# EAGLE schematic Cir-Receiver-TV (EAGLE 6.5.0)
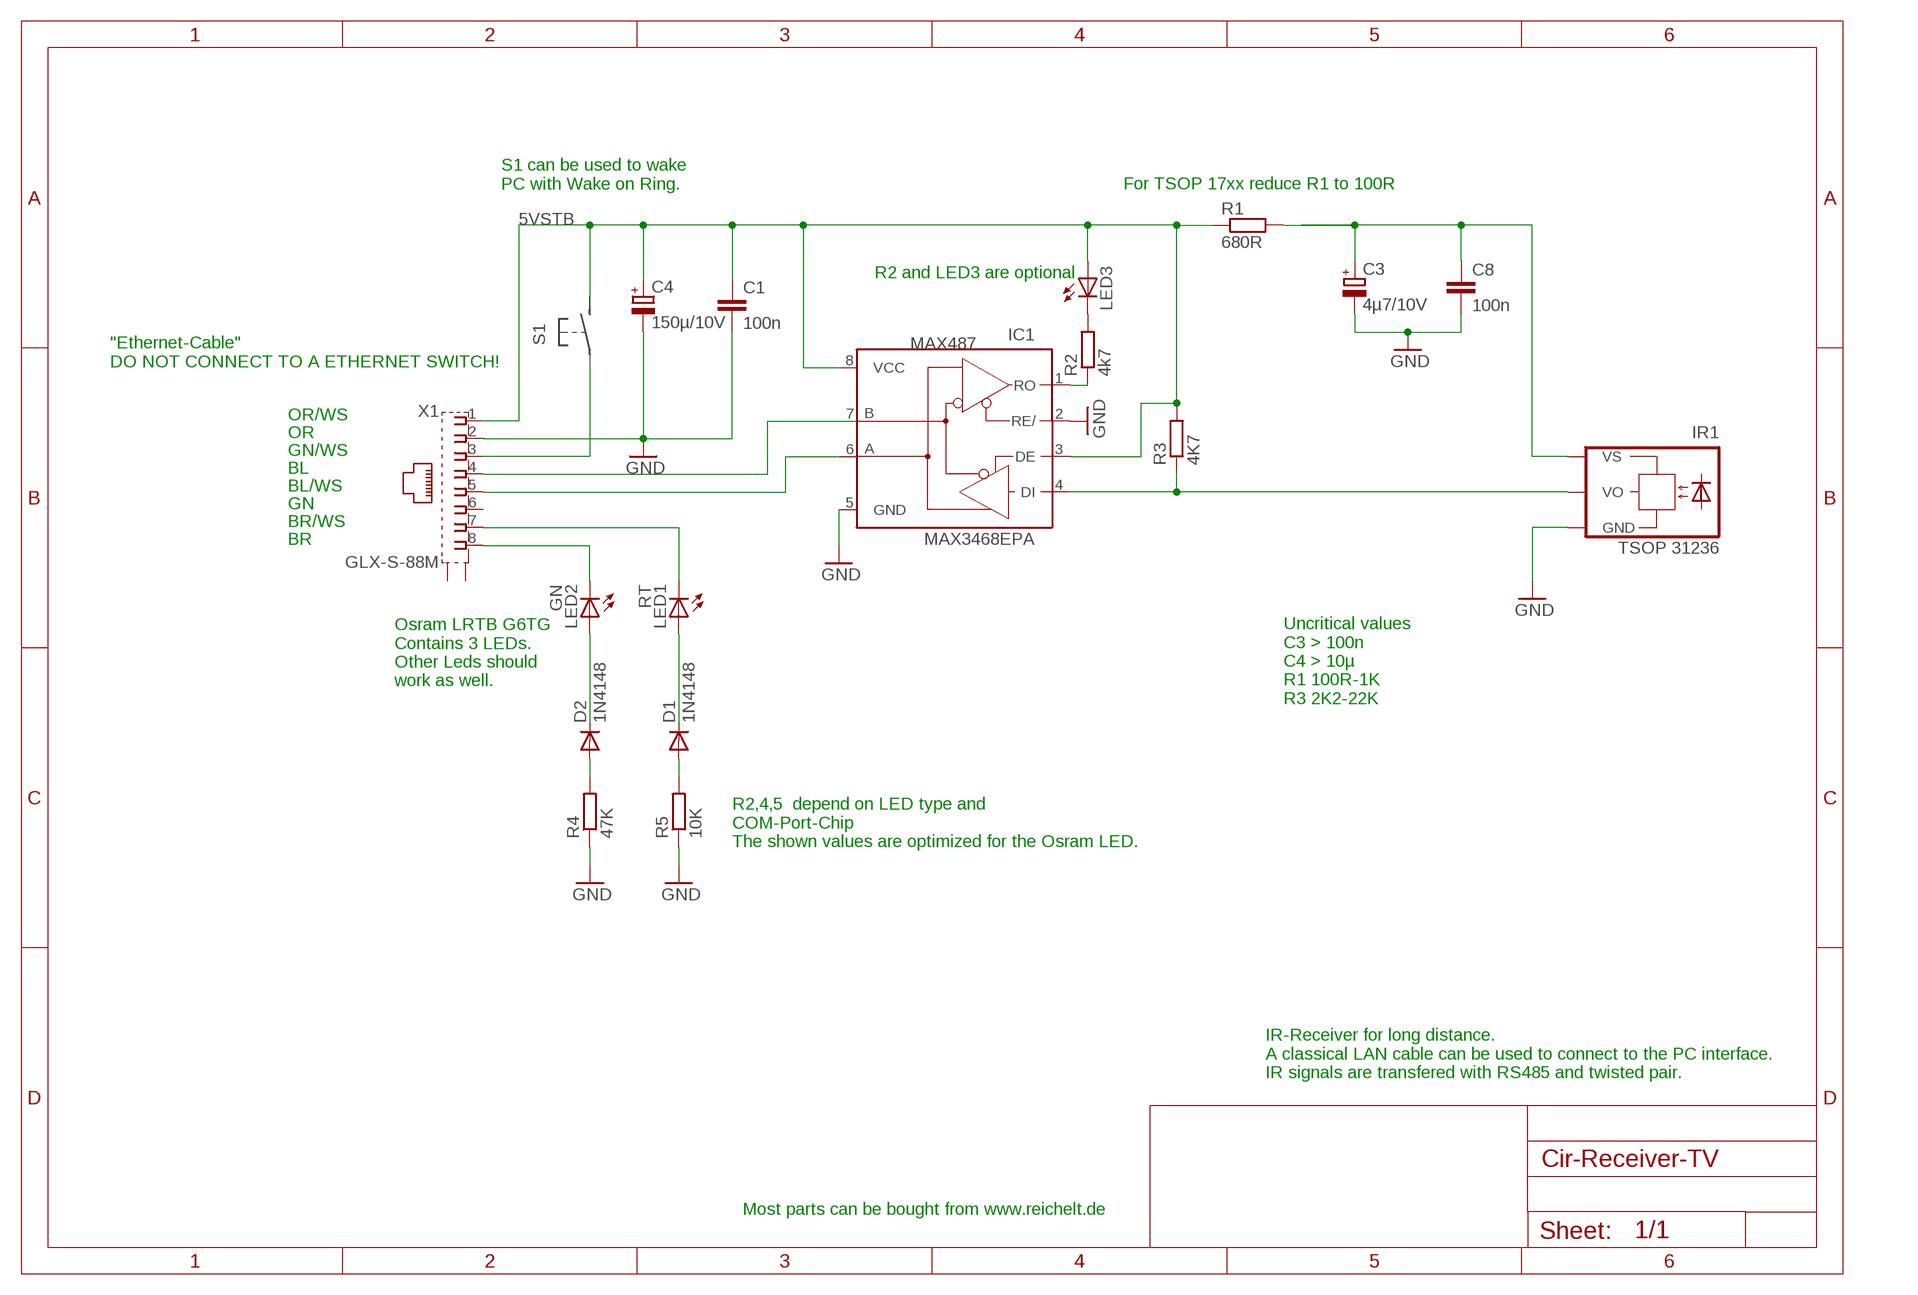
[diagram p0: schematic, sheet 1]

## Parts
C1  100n  C2,5-3  [C2.5-3]
C3  4µ7/10V  CPOL-EUE2.5-5  [E2,5-5]
C4  150µ/10V  CPOL-EUE2.5-5  [E2,5-5]
C8  100n  C2,5-3  [C2.5-3]
D1  1N4148  1N4148DO35-7  [DO35-7]
D2  1N4148  1N4148DO35-7  [DO35-7]
IC1  MAX3468EPA  [DIL08]
IR1  TSOP 31236  TSOP1737TB1  [TSOP17_TB1]
LED1  RT  LED3MM  [LED3MM]
LED2  GN  LED3MM  [LED3MM]
LED3  LED3MM  [LED3MM]
R1  680R  R-EU_0207/10  [0207/10]
R2  4k7  R-EU_0207/10  [0207/10]
R3  4K7  R-EU_0207/10  [0207/10]
R4  47K  R-EU_0207/10  [0207/10]
R5  10K  R-EU_0207/10  [0207/10]
X1  GLX-S-88M  [GLX-S-88M]

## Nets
5VSTB: C1.1 C4.+ IC1.3(DE) IC1.8(VCC) LED3.A R1.1 R3.2 X1.1
GND: C1.2 C3.- C4.- C8.2 IC1.2(RE/) IC1.5(GND) IR1.GND R4.1 R5.1 X1.2
N$1: C3.+ C8.1 IR1.VS R1.2
N$2: IC1.4(DI) IR1.VO R3.1
N$3: X1.3
N$4: LED3.K(C) R2.2
N$5: IC1.1(RO) R2.1
N$6: D1.A R5.2
N$7: IC1.7(B) X1.4
N$8: IC1.6(A) X1.5
N$9: D2.A R4.2
N$10: D1.C LED1.A
N$11: LED2.K(C) X1.8
N$12: LED1.K(C) X1.7
N$13: D2.C LED2.A
Unconnected: X1.6 X1.S1 X1.S2

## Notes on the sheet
- S1 can be used to wake
  PC with Wake on Ring.
- For TSOP 17xx reduce R1 to 100R
- R2 and LED3 are optional
- "Ethernet-Cable"
  DO NOT CONNECT TO A ETHERNET SWITCH!
- OR/WS
- OR
- GN/WS
- BL
- BL/WS
- GN
- BR/WS
- BR
- Osram LRTB G6TG
  Contains 3 LEDs.
  Other Leds should
  work as well.
- Uncritical values
  C3 > 100n
  C4 > 10µ
  R1 100R-1K
  R3 2K2-22K
- R2,4,5  depend on LED type and
  COM-Port-Chip
  The shown values are optimized for the Osram LED.
- IR-Receiver for long distance.
  A classical LAN cable can be used to connect to the PC interface.
  IR signals are transfered with RS485 and twisted pair.
- Most parts can be bought from www.reichelt.de

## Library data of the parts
C1 C8 = capacitor-wima:C: CAPACITOR
C3 C4 = rcl:CPOL-EU: POLARIZED CAPACITOR, European symbol
D1 D2 = diode:1N4148: DIODE
IC1 = maxim:MAX34*: +5V, Fail-Safe, 40Mbps, Profibus RS-485/RS-422 Transceivers Source: MAX3465-MAX3469.pdf; MPN: MAX487; OC_FARNELL: unknown
IR1 = telefunken:TSOP17*TB1: TSOP17..TB1 IR Receiver Modules for Remote Control Systems Source: http://www.vishay.com/docs/82042/82042.pdf; OC_FARNELL: unknown; OC_NEWARK: unknown
LED1-LED3 = led:LED: LED
R1-R5 = resistor:R-EU_: RESISTOR, European symbol
X1 = con-kycon:GLX-S-88M: Mod. Jack, Right Angle, 8 posiotion, 8 contatcs RJ45 Source: GLX-S-88M.pdf; OC_FARNELL: unknown; OC_NEWARK: unknown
